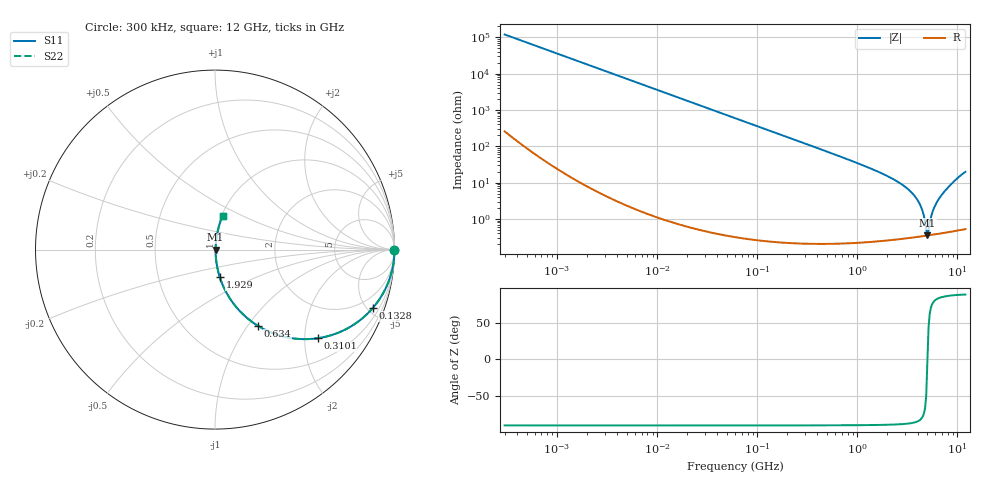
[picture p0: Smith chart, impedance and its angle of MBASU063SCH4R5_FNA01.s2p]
! MBASU063SCH4R5_FNA01  S-PARAMETER MODEL  ( General Type )
! Model Generated by TAIYO YUDEN Corporation (http://www.ty-top.com)
! Version 1.0
! TAIYO YUDEN Control No. 130801
! Copyright(c) 2013 TAIYO YUDEN CO.,LTD. All Rights Reserved.
! Product Description (link to TY-COMPAS)
! https://ds.yuden.co.jp/TYCOMPAS/or/detail?pn=MBASU063SCH4R5CFNA01&u=M
! Products Name : Multilayer Ceramic Capacitors
! Characteristics :
!  Capacitance : 4.5 pF , Rated Voltage : 50V , TCC : CH / C0H
!  Case Size : 0.6 x 0.3 / 0.024 x 0.012 [mm/inch] , Thickness : 0.3 / 0.012 [mm/inch]
!  (Conditions: Temperature = 25 degC , DC Bias Current/Voltage = 0A / 0V)
! External Node Assignments :
!  1  o---| |---o  2
! GND o---------o GND
! Frequency Range : 0.3MHz  -  12000MHz  [ 401 STEP ]
# MHz S RI R 50
! Freq[MHz].  S11 Real  S11 Imag  S21 Real  S21 Imag  S12 Real  S12 Imag  S22 Real  S22 Imag
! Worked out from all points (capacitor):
!   401 points, 300 kHz to 12 GHz, reference 50 ohm
!   read as one part in series: C = 4.43 pF near 316.3 kHz
!   lowest |Z| = 351 mohm at 5.006 GHz (marker M1)
!   series resonance near 5.014 GHz, so ESL is about 230 pH
!   S11 on the Smith chart (normalised r, x): 300 kHz: open; 132.8 MHz: 1.00, -5.41; 310.1 MHz: 1.00, -2.31; 634 MHz: 1.00, -1.12; 1.929 GHz: 1.01, -0.32; 12 GHz: 1.01, +0.40
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0.3  1 -0.000835  2.49e-06 0.000835  2.49e-06 0.000835  1 -0.000835
1.769972  1 -0.00493  2.66e-05 0.00493  2.66e-05 0.00493  1 -0.00493
10.44266  0.9991 -0.029  0.000853 0.029  0.000853 0.029  0.9991 -0.029
60  0.9728 -0.1625  0.0272 0.1625  0.0272 0.1625  0.9728 -0.1625
132.8329  0.8794 -0.3252  0.1206 0.3252  0.1206 0.3252  0.8794 -0.3252
310.0777  0.5711 -0.494  0.4289 0.494  0.4289 0.494  0.5711 -0.494
353.9943  0.5049 -0.499  0.4951 0.499  0.4951 0.499  0.5049 -0.499
634.0297  0.238 -0.424  0.762 0.424  0.762 0.424  0.238 -0.424
1048.836  0.0985 -0.2946  0.9015 0.2946  0.9015 0.2946  0.0985 -0.2946
1928.972  0.0269 -0.154  0.9731 0.154  0.9731 0.154  0.0269 -0.154
2088.533  0.0222 -0.1386  0.9778 0.1386  0.9778 0.1386  0.0222 -0.1386
2947.191  0.00914 -0.0788  0.9909 0.0788  0.9909 0.0788  0.00914 -0.0788
3740.715  0.00491 -0.0422  0.9951 0.0422  0.9951 0.0422  0.00491 -0.0422
4270.516  0.0038 -0.0229  0.9962 0.0229  0.9962 0.0229  0.0038 -0.0229
4502.883  0.00358 -0.0153  0.9964 0.0153  0.9964 0.0153  0.00358 -0.0153
4875.354  0.00347 -0.00397  0.9965 0.00397  0.9965 0.00397  0.00347 -0.00397
5006.236  0.00349 -0.000209  0.9965 0.000209  0.9965 0.000209  0.00349 -0.000209
5278.635  0.00361 0.00659  0.9964 -0.00659  0.9964 -0.00659  0.00361 0.00659
5868.704  0.00415 0.0204  0.9959 -0.0204  0.9959 -0.0204  0.00415 0.0204
6699.894  0.0055 0.0392  0.9945 -0.0392  0.9945 -0.0392  0.0055 0.0392
8966.534  0.0143 0.0979  0.9857 -0.0979  0.9857 -0.0979  0.0143 0.0979
12000  0.0424 0.1887  0.9576 -0.1887  0.9576 -0.1887  0.0424 0.1887
